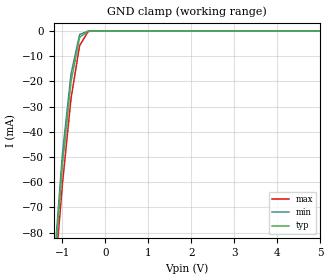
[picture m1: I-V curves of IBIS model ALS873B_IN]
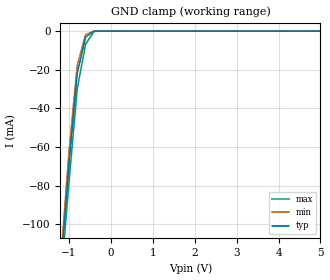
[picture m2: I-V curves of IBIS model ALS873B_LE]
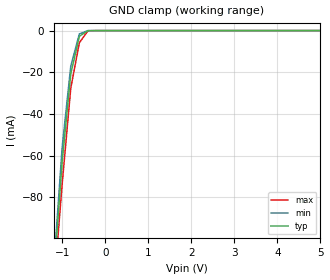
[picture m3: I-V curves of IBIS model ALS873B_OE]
|   TEXAS INSTRUMENTS INCORPORATED
|   Standard Linear and Logic Group
|   IBIS Model of SN74ALS873B
|   DUAL 4-BIT D-TYPE LATCHES WITH 3-STATE OUTPUTS
|   DIP 24-pin (NT), SOL 24-pin (DW)
[IBIS Ver]   3.2
[Comment char] |_char
[File Name]   sn74als873b.ibs
[File Rev]   1.1 | c_die
[Date]   Mar 10,2004
[Source]   File originated at Texas Instruments, Inc
[Notes]   The following is a sample IBIS file for the SN74ALS873B.
   - FILE REV HISTORY
   - 1.1 Release IBIS file on 03/17/04
   - Power clamp data deleted as there is no power-clamp diode.
|   - All test data contained in this file are derived from
|   actual measurement.
|   - The measurement used DW package.
|   - We have data across voltage and temperature, but not across
|   process.
|   - We have some end-point warnings due to 50 ohms load
|   for ac data
[Disclaimer] Property of Texas Instruments Incorporated.  Unauthorized
   reproduction and/or distribution is strictly prohibited.
   This product is protected under copyright law.
   Created  2002, (C) Copyright  2002, Texas Instruments
   Incorporated, All Rights Reserved
   UNLESS THERE IS A SIGNED, WRITTEN AGREEMENT TO THE
   CONTRARY, TEXAS INSTRUMENTS (TI) IS PROVIDING THE IBIS
   MODELS  AND WITHOUT ANY WARRANTY, EXPRESSED OR
   IMPLIED.  TI assumes no liability for:
   1) the accuracy of the IBIS models provided to your
   company;
   2) the proper functioning of these IBIS Models in your
   design or for any resulting applications; or
   3) infringement of patents, copyrights or intellectual
   property rights resulting from your use of these IBIS
   models.
   TI provides IBIS Models as a service to our customers.
   You and your company shall not distribute, sell or give
   these models to anyone else without prior written
   permission from TI.
   TI reserves the right to make changes to our products or
   to discontinue any semiconductor product or service
   without notice, and advises our customers to obtain the
   latest version of relevant information to verify, before
   placing orders, that the information being relied on is
   current.
   Please be aware that your receipt and use of the IBIS
   information provided shall serve as acceptance of these
   terms and conditions.  If you do not accept these terms,
   you should return or destroy the IBIS models and any
   other accompanying information immediately.
|   Component SN74ALS873B_NT
[Component]   SN74ALS873B_NT
[Manufacturer]  Texas Instruments, Inc.
[Package]
|   typ   min   max
R_pkg   0.057   0.039   0.068
L_pkg   8.201nH   4.977nH   13.831nH
C_pkg   1.359pF   0.776pF   2.368pF
[Pin]   signal_name   model_name   R_pin   L_pin   C_pin
1   1CLR_BAR   ALS873B_CLR   0.050   11.787nH   1.945pF
2   1OE_BAR   ALS873B_OE   0.055   10.061nH   1.944pF
3   1D1   ALS873B_IN   0.064   8.944nH   1.402pF
4   1D2   ALS873B_IN   0.068   8.005nH   1.041pF
5   1D3   ALS873B_IN   0.059   5.529nH   0.801pF
6   1D4   ALS873B_IN   0.058   4.977nH   1.008pF
7   2D1   ALS873B_IN   0.058   4.977nH   1.010pF
8   2D2   ALS873B_IN   0.059   5.527nH   0.780pF
9   2D3   ALS873B_IN   0.052   7.906nH   1.058pF
10   2D4   ALS873B_IN   0.052   8.855nH   1.437pF
11   2OE_BAR   ALS873B_OE   0.055   12.114nH   2.334pF
12   GND   GND   0.063   13.831nH   2.368pF
13   2CLR_BAR   ALS873B_CLR   0.063   11.817nH   1.927pF
14   2LE   ALS873B_LE   0.056   10.120nH   1.888pF
15   2Q4   ALS873B_OUT   0.054   8.837nH   1.438pF
16   2Q3   ALS873B_OUT   0.052   7.790nH   1.261pF
17   2Q2   ALS873B_OUT   0.059   5.415nH   0.981pF
18   2Q1   ALS873B_OUT   0.058   5.090nH   0.802pF
19   1Q4   ALS873B_OUT   0.058   5.097nH   0.802pF
20   1Q3   ALS873B_OUT   0.059   5.529nH   0.776pF
21   1Q2   ALS873B_OUT   0.052   7.838nH   1.057pF
22   1Q1   ALS873B_OUT   0.039   8.783nH   1.446pF
23   1LE   ALS873B_LE   0.059   8.101nH   1.556pF
24   VCC   POWER   0.062   9.883nH   1.550pF
|   Component SN74ALS873B_DW
[Component]   SN74ALS873B_DW
[Manufacturer]  Texas Instruments, Inc.
[Package]
|   typ   min   max
R_pkg   0.037   0.030   0.047
L_pkg   5.146nH   3.993nH   6.885nH
C_pkg   0.758pF   0.512pF   1.067pF
[Pin]   signal_name   model_name   R_pin   L_pin   C_pin
1   1CLR_BAR   ALS873B_CLR   0.039   6.885nH   1.067pF
2   1OE_BAR   ALS873B_OE   0.042   5.950nH   0.958pF
3   1D1   ALS873B_IN   0.047   5.317nH   0.791pF
4   1D2   ALS873B_IN   0.031   4.651nH   0.611pF
5   1D3   ALS873B_IN   0.030   3.993nH   0.512pF
6   1D4   ALS873B_IN   0.030   4.083nH   0.611pF
7   2D1   ALS873B_IN   0.030   4.083nH   0.611pF
8   2D2   ALS873B_IN   0.030   3.993nH   0.512pF
9   2D3   ALS873B_IN   0.031   4.652nH   0.611pF
10   2D4   ALS873B_IN   0.047   5.317nH   0.791pF
11   2OE_BAR   ALS873B_OE   0.042   5.950nH   0.959pF
12   GND   GND   0.039   6.885nH   1.067pF
13   2CLR_BAR   ALS873B_CLR   0.039   6.885nH   1.067pF
14   2LE   ALS873B_LE   0.042   5.950nH   0.959pF
15   2Q4   ALS873B_OUT   0.047   5.317nH   0.791pF
16   2Q3   ALS873B_OUT   0.031   4.652nH   0.611pF
17   2Q2   ALS873B_OUT   0.030   3.993nH   0.512pF
18   2Q1   ALS873B_OUT   0.030   4.083nH   0.610pF
19   1Q4   ALS873B_OUT   0.030   4.083nH   0.610pF
20   1Q3   ALS873B_OUT   0.030   3.993nH   0.512pF
21   1Q2   ALS873B_OUT   0.031   4.651nH   0.611pF
22   1Q1   ALS873B_OUT   0.047   5.317nH   0.791pF
23   1LE   ALS873B_LE   0.042   5.950nH   0.958pF
24   VCC   POWER   0.039   6.885nH   1.067pF
| Models and submodels in the file (5): ALS873B_IN (Input), ALS873B_LE (Input), ALS873B_OE (Input), ALS873B_CLR (Input), ALS873B_OUT (3-state)
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|   Model ALS873B_IN
[Model]   ALS873B_IN
Model_type  Input
Polarity   Non-Inverting
Vinl = 0.8
Vinh = 2.0
| variable   typ   min   max
C_comp   4.889pf   4.865pf   4.961pf
[Temperature Range]   25   0   70
[Voltage Range]   5.0   4.5   5.5
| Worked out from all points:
|   GND clamp passes 1 mA (typ) near -0.48 V on its own axis
[GND Clamp]
|   Voltage   I(typ)   I(min)   I(max)
-5V       -1.162A    -1.229A    -1.045A
-1.2V     -97.27mA   -94.03mA   -102.4mA
-1V       -53.11mA   -48.81mA   -60.75mA
-800mV    -20.04mA   -17.02mA   -26.75mA
-600mV    -2.453mA   -1.329mA   -5.754mA
-400mV    -14.77uA   -7.304uA   -110.6uA
5V        5.06pA     7.54pA     166.5pA
|   Model ALS873B_LE
[Model]   ALS873B_LE
Model_type  Input
Polarity   Non-Inverting
Vinl = 0.8
Vinh = 2.0
| variable   typ   min   max
C_comp   5.126pf   5.097pf   5.174pf
[Temperature Range]   25   0   70
[Voltage Range]   5.0   4.5   5.5
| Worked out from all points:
|   GND clamp passes 1 mA (typ) near -0.46 V on its own axis
[GND Clamp]
|   Voltage   I(typ)   I(min)   I(max)
-5V       -1.49A     -1.551A    -1.354A
-1.2V     -125.3mA   -120.6mA   -132mA
-1V       -70.05mA   -63.26mA   -79.24mA
-800mV    -21.87mA   -17.82mA   -29.95mA
-600mV    -3.12mA    -1.81mA    -6.749mA
-400mV    -29.78uA   -16.03uA   -201.2uA
5V        6.76pA     10.24pA    266.3pA
|   Model ALS873B_OE
[Model]   ALS873B_OE
Model_type  Input
Polarity   Inverting
Vinl = 0.8
Vinh = 2.0
| variable   typ   min   max
C_comp   5.199pf   5.170pf   5.258pf
[Temperature Range]   25   0   70
[Voltage Range]   5.0   4.5   5.5
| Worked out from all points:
|   GND clamp passes 1 mA (typ) near -0.47 V on its own axis
[GND Clamp]
|   Voltage   I(typ)   I(min)   I(max)
-5V       -1.308A    -1.362A    -1.217A
-1.2V     -119.6mA   -115.3mA   -125.5mA
-1V       -63.01mA   -56.17mA   -73.82mA
-800mV    -20.83mA   -17.13mA   -27.73mA
-600mV    -2.73mA    -1.604mA   -5.839mA
-400mV    -24.48uA   -14.94uA   -131.4uA
5V        23.24pA    14.78pA    205.3pA
